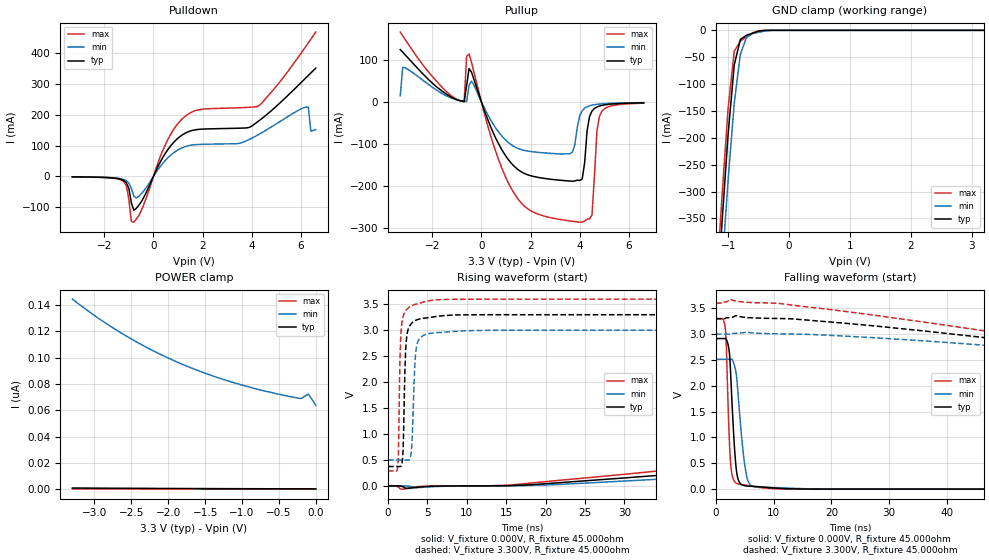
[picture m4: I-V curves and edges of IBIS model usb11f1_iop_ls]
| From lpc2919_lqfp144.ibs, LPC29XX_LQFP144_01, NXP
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| usb11f1
|   Universal Serial Bus Pad
|   Revision 1.1 Specification
|   Programmable Single Ended Core Input
|   Forced Single Ended Low
|   Switchable between
|   - high speed output mode
|   - low speed output mode
|   - low/high speed input mode
| |   Rev 0.20 IBIS Model Design Automation Generation   |
| |   N O N - S I L I C O N   C O R R E L A T E D   |
| |   This IBIS [Model] is pre-Beta tactical support   |
| |  Note: this IBIS [Model] contains clamp curves generated   |
| |   through simulation which should not be relied upon   |
| Pccmos14 hliolib_nlm 4.0
|   0.18 um 3.3V pad library
|   six level metal
|   dual oxide
|   single threshold voltage
|   nominal line mixed supply
|   parasitic extracted netlists
| Process block c14
| Low Speed Output Mode
[Model]   usb11f1_iop_ls | of usb11f1
Model_type   I/O
Polarity   Non-Inverting
Enable   Active-Low
|  Reciever Thresholds
Vinl   = 0.8V
Vinh   = 2.0V
| AC Test Load Conditions
Vref   = 0
Cref   = 0
Rref   = 1000000000
Vmeas   = 1.65
| [Process Range]   typical   min   max
| C_comp edge width   400.000ps   400.000ps   400.000ps
| C_comp Tstrobe   40.000fs   40.000fs   40.000fs
C_comp   3.752pF   3.496pF   4.045pF
[Temperature Range]   25   125   -40
[Voltage Range]   3.30V   3.00V   3.60V
[GND Clamp Reference]   0.00V   0.00V   0.00V
[Pulldown Reference]   0.00V   0.00V   0.00V
[POWER Clamp Reference]   3.30V   3.00V   3.60V
[Pullup Reference]   3.30V   3.00V   3.60V
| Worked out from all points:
|   slope of the pulldown table from 0 to 0.495 V, typ, clamps not added: 6.48 ohm
|   slope of the pullup table from 0 to 0.495 V, typ, clamps not added: 6.61 ohm
|   GND clamp passes 1 mA (typ) near -0.46 V on its own axis
|   rising waveform, V_fixture 0.000V, R_fixture 45.000ohm: 20-80 % time 151ns typ, 180ns min, 132ns max; typ from 0 V to 2.91 V
|   falling waveform, V_fixture 0.000V, R_fixture 45.000ohm: 20-80 % time 849ps typ, 1.23ns min, 610ps max; typ from 2.91 V to 0 V
|   rising waveform, V_fixture 3.300V, R_fixture 45.000ohm: 20-80 % time 319ps typ, 398ps min, 283ps max; typ from 0.374 V to 3.3 V
|   falling waveform, V_fixture 3.300V, R_fixture 45.000ohm: 20-80 % time 156ns typ, 194ns min, 133ns max; typ from 3.3 V to 0.38 V
[GND Clamp]
| ref voltage   0.00V   0.00V   0.00V
|   Voltage   I(typ)   I(min)   I(max)
-3.3V     -4.618A    -4.67A     -4.591A
-1.2V     -533.4mA   -616mA     -486.2mA
-1.1V     -356.1mA   -441.1mA   -306.9mA
-1V       -192.1mA   -277.1mA   -143.8mA
-900mV    -64.59mA   -135.6mA   -38.91mA
-800mV    -17.04mA   -44.51mA   -19.95mA
-700mV    -9.237mA   -13.86mA   -12.52mA
-600mV    -5.456mA   -6.064mA   -4.789mA
-500mV    -1.495mA   -3.666mA   -840.2uA
-300mV    -6.625uA   -179.7uA   -408.9nA
3.2V      293.2pA    68.89nA    105.6pA
[Power Clamp]   | Vtable = Vcc - Vpad
| ref voltage   3.30V   3.00V   3.60V
|   Voltage   I(typ)   I(min)   I(max)
-3.3V     1.005nA    144.5nA    354.7pA
-3V       911.2pA    132nA      335.1pA
-2.6V     800.8pA    117.4nA    309pA
-2.3V     727.5pA    108nA      289.6pA
-1.9V     640.7pA    97.15nA    263.8pA
-1.6V     582.9pA    90.25nA    244.5pA
-1.3V     530.6pA    84.3nA     225.3pA
-1V       483pA      79.18nA    206.1pA
-700mV    439.6pA    74.79nA    187pA
-200mV    377.6pA    68.89nA    155pA
-100mV    416.5pA    72.39nA    142.6pA
0V        319.1pA    63.83nA    125.6pA
[Pulldown]
| ref voltage   0.00V   0.00V   0.00V
|   Voltage   I(typ)   I(min)   I(max)
-3.3V     -1.652mA   -1.454mA   -1.796mA
-1.2V     -13.92mA   -10.45mA   -17.73mA
-1.1V     -21.12mA   -14.45mA   -30.61mA
-900mV    -85.23mA   -38.63mA   -146.6mA
-800mV    -110mA     -63.62mA   -148.7mA
500mV     77.03mA    53.28mA    105.7mA
1.1V      130.5mA    90.36mA    180.9mA
4.3V      181mA      136.8mA    229.8mA
6.2V      319.7mA    225.1mA    421.9mA
6.3V      327.6mA    224.1mA    433.3mA
6.4V      335.5mA    146.8mA    444.9mA
6.6V      351.2mA    151.8mA    468.2mA
[Pullup]   | Vtable = Vcc - Vpad
| ref voltage   3.30V   3.00V   3.60V
|   Voltage   I(typ)   I(min)   I(max)
-3.3V     123.9mA    14.28mA    165.4mA
-3.2V     117.8mA    81.84mA    156.7mA
-800mV    1.807mA    2.206mA    1.368mA
-500mV    79.1mA     39.57mA    113.5mA
1V        -129mA     -91.21mA   -180.1mA
2.5V      -180.9mA   -120.7mA   -269.8mA
3.7V      -188.1mA   -119.1mA   -283mA
4.1V      -182.9mA   -20.96mA   -285.2mA
4.4V      -34.22mA   -9.287mA   -277.5mA
4.5V      -21.68mA   -7.778mA   -267.6mA
4.8V      -9.883mA   -5.195mA   -34.66mA
6.6V      -2.365mA   -1.804mA   -3.161mA
[Ramp]
R_load   = 60.000ohm
|   dV/dt(typ)   dV/dt(min)   dV/dt(max)
dV/dt_r   621.190mV/49.000ns   449.928mV/47.650ns   797.802mV/50.350ns
dV/dt_f   625.429mV/49.850ns   419.411mV/47.250ns   836.564mV/52.050ns
[Rising Waveform]  | cubic spline decimation from 16001 points
V_fixture   = 0.000V
R_fixture   = 45.000ohm
|   Time   V(typ)   V(min)   V(max)
0s        443.9pV    34.49nV    250.2pV
1.75ns    -12.44mV   -77.09nV   -62.9mV
15.7ns    6.216mV    2.653mV    19.45mV
132.3ns   1.434V     1.053V     1.828V
189ns     2.07V      1.539V     2.618V
215ns     2.322V     1.74V      2.889V
240ns     2.51V      1.913V     3.03V
309.8ns   2.74V      2.231V     3.186V
379.5ns   2.823V     2.359V     3.238V
800ns     2.907V     2.501V     3.292V
[Falling Waveform]  | cubic spline decimation from 2001 points
V_fixture   = 0.000V
R_fixture   = 45.000ohm
|   Time   V(typ)   V(min)   V(max)
0s        2.914V     2.514V     3.296V
1.6ns     2.916V     2.514V     3.122V
1.75ns    2.906V     2.514V     2.897V
2.25ns    2.702V     2.514V     1.129V
2.75ns    1.732V     2.515V     298mV
3.35ns    581.4mV    2.329V     131.3mV
3.9ns     170mV      1.737V     97.45mV
5.3ns     61.74mV    255.6mV    74.9mV
6.8ns     52.46mV    46.91mV    45.36mV
100ns     89.64uV    121.6uV    67.51uV
[Rising Waveform]  | cubic spline decimation from 2001 points
V_fixture   = 3.300V
V_fixture_min = 3.000V
V_fixture_max = 3.600V
R_fixture   = 45.000ohm
|   Time   V(typ)   V(min)   V(max)
0s        373.7mV    499.4mV    287.7mV
1.25ns    373.7mV    499.5mV    413.6mV
1.55ns    374.7mV    499.5mV    2.639V
1.85ns    543.1mV    499.5mV    3.228V
2.2ns     2.498V     499.5mV    3.365V
2.45ns    2.956V     499.6mV    3.412V
3ns       3.135V     750.5mV    3.472V
3.6ns     3.196V     2.669V     3.504V
5.1ns     3.242V     2.932V     3.564V
100ns     3.3V       3V         3.6V
[Falling Waveform]  | cubic spline decimation from 16001 points
V_fixture   = 3.300V
V_fixture_min = 3.000V
V_fixture_max = 3.600V
R_fixture   = 45.000ohm
|   Time   V(typ)   V(min)   V(max)
0s        3.3V       3V         3.6V
2.45ns    3.319V     3V         3.678V
21.65ns   3.217V     2.965V     3.45V
110.3ns   2.131V     2.208V     2.045V
178.1ns   1.363V     1.644V     1.065V
209.7ns   1.051V     1.407V     708.1mV
234.1ns   848.5mV    1.239V     550.7mV
304.6ns   556mV      858.2mV    387.2mV
389.8ns   453.6mV    659.6mV    332.3mV
800ns     380mV      513mV      291.2mV
